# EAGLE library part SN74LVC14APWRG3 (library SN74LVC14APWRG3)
Hex Schmitt-Trigger Inverter Source: Datasheet
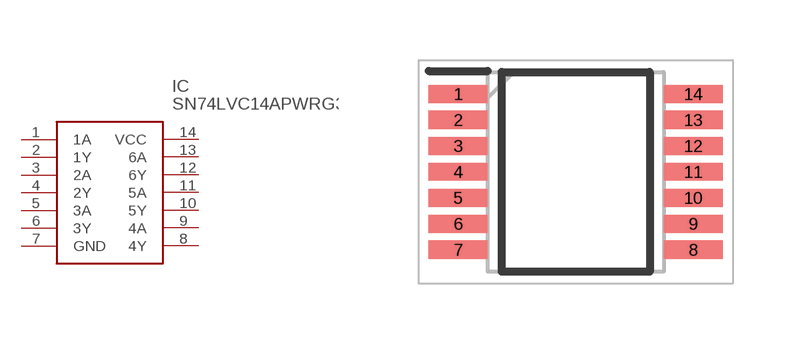
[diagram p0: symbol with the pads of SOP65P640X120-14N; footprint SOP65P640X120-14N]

Designator prefix IC

## SN74LVC14APWRG3 (Description: Hex Schmitt-Trigger Inverter; Height: 1.2mm; Manufacturer_Name: Texas Instruments; Manufacturer_Part_Number: SN74LVC14APWRG3; Mouser_Part_Number: 595-SN74LVC14APWRG3; Mouser_Price-Stock: https://www.mouser.co.uk/ProductDetail/Texas-Instruments/SN74LVC14APWRG3?qs=GI4%2FryNtbd0oVXocaK57NQ%3D%3D)  [SOP65P640X120-14N]
1  1A
2  1Y
3  2A
4  2Y
5  3A
6  3Y
7  GND
8  4Y
9  4A
10  5Y
11  5A
12  6Y
13  6A
14  VCC

## Footprint SOP65P640X120-14N (pad centres in mm)
PW
smd 1.475 x 0.45: 1 -2.938,1.95; 2 -2.938,1.3; 3 -2.938,0.65; 4 -2.938,0; 5 -2.938,-0.65; 6 -2.938,-1.3; 7 -2.938,-1.95; 8 2.938,-1.95; 9 2.938,-1.3; 10 2.938,-0.65; 11 2.938,0; 12 2.938,0.65; 13 2.938,1.3; 14 2.938,1.95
